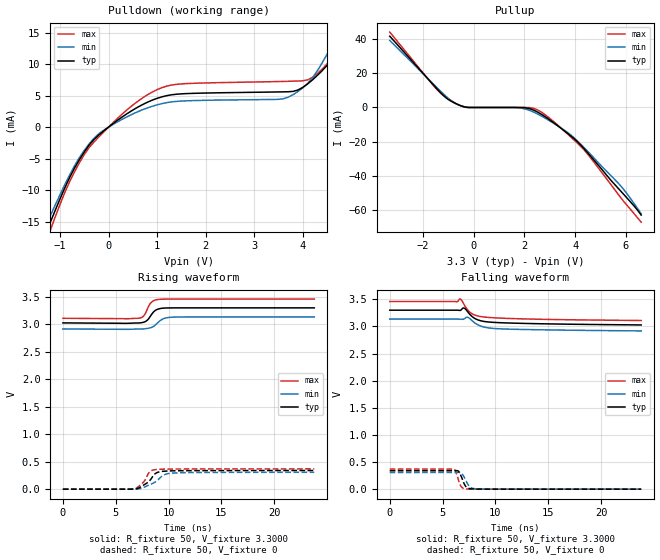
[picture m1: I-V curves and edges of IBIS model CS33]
|   IBIS Models For TG-5511CA (ClippedSine)
[IBIS Ver]   3.2
[File name]   tg5511ca_cs.ibs
[File Rev]   1.0
[Date]   Dec 3, 2020
[Source]   From silicon level SPICE model at Seiko Epson.
[Notes]
[Disclaimer]
This information is for modeling purposes only, and is not guaranteed.
Property of SEIKO EPSON Corp.,
unauthorized reproduction and/or distribution is strictly prohibited.
[Copyright]   Copyright 2020, SEIKO EPSON Corp. All rights reserved.
[Component]   TG-5511CA (ClippedSine)
[Manufacturer] SEIKO EPSON Corp.
[Package]
| variable   typ   min   max
R_pkg   99.0m   NA   NA
L_pkg   3.29n   NA   NA
C_pkg   0.40p   NA   NA
[Pin] signal_name   model_name   R_pin  L_pin  C_pin
  2   GND   GND   NA   NA   NA
  3   OUT   CS33   NA   NA   NA
  4   VCC   POWER   NA   NA   NA
| Models and submodels in the file (1): CS33 (Output)
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|   Model_type Output
[Model] CS33
Model_type  Output
Enable   Active-High
Polarity   Non-Inverting
Vmeas = 1.65
C_comp   2.5p   2.0p   3.0p
[Temperature Range]   25   85   -40
[Voltage Range]   3.3000   3.1350   3.4650
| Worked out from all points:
|   slope of the pulldown table from 0 to 0.495 V, typ, clamps not added: 184 ohm
|   falling waveform, R_fixture 50, V_fixture 3.3000: 20-80 % time 1.88ns typ, 2.1ns min, 1.61ns max; typ from 3.3 V to 3.03 V
|   falling waveform, R_fixture 50, V_fixture 0: 20-80 % time 453ps typ, 527ps min, 385ps max; typ from 0.34 V to 0 V
|   rising waveform, R_fixture 50, V_fixture 3.3000: 20-80 % time 675ps typ, 839ps min, 578ps max; typ from 3.03 V to 3.3 V
|   rising waveform, R_fixture 50, V_fixture 0: 20-80 % time 1.09ns typ, 1.46ns min, 815ps max; typ from 0 V to 0.34 V
[Pullup]
|   voltage I(typ)   I(min)   I(max)
-3.3V     41.62mA    39.12mA    44.01mA
-1.4V     10.28mA    11.01mA    9.827mA
-1.1V     5.864mA    6.748mA    6.095mA
-700mV    2.283mA    2.267mA    2.407mA
-300mV    152.5uA    251.6uA    75.7uA
1.8V      -4.05uA    -213.2uA   -94.5pA
2.3V      -1.159mA   -2.247mA   -272.4uA
2.8V      -5.195mA   -6.055mA   -4.027mA
3.7V      -15.1mA    -14.57mA   -15.44mA
4.2V      -21.6mA    -21.15mA   -22.42mA
5.8V      -48.88mA   -45.87mA   -52.72mA
6.6V      -62.82mA   -61.97mA   -66.95mA
[Pulldown]
|   voltage I(typ)   I(min)   I(max)
-3.3V     -61.57mA   -57.79mA   -65.45mA
-1.4V     -18.98mA   -17.58mA   -20.64mA
-1.2V     -15.12mA   -14.09mA   -16.38mA
-700mV    -6.498mA   -6.139mA   -7.097mA
-300mV    -1.962mA   -1.771mA   -2.366mA
1V        4.571mA    3.539mA    5.95mA
3.6V      5.603mA    4.498mA    7.258mA
4.2V      7.484mA    7.785mA    7.888mA
4.8V      13.35mA    15.8mA     12.77mA
5V        16.43mA    18.73mA    14.85mA
5.1V      18.03mA    20.21mA    16.09mA
6.6V      42.74mA    42.3mA     42.63mA
[Falling Waveform]
R_fixture = 50
V_fixture = 3.3000
V_fixture_min = 3.1350
V_fixture_max = 3.4650
0s        3.3V       3.135V     3.46V
6.4ns     3.3V       3.135V     3.455V
6.7ns     3.297V     3.134V     3.505V
6.9ns     3.336V     3.131V     3.454V
7.1ns     3.333V     3.146V     3.384V
7.4ns     3.265V     3.168V     3.299V
7.7ns     3.199V     3.124V     3.245V
8.4ns     3.117V     3.024V     3.19V
9.4ns     3.082V     2.972V     3.166V
23.8ns    3.028V     2.918V     3.11V
[Falling Waveform]
R_fixture = 50
V_fixture = 0
V_fixture_min = 0
V_fixture_max = 0
0s        340mV      307.6mV    370mV
6.1ns     340.9mV    308.7mV    369.9mV
6.2ns     341mV      308.7mV    347.7mV
6.5ns     333mV      308.7mV    173.9mV
6.7ns     264.1mV    304.2mV    66.64mV
6.9ns     171.9mV    269.7mV    22.06mV
7.2ns     49.75mV    165.3mV    5.263mV
7.6ns     8.533mV    41.6mV     1.957mV
8.3ns     1.868mV    5.22mV     789.2uV
23.8ns    0V         219.5uV    0V
[Rising Waveform]
R_fixture = 50
V_fixture = 3.3000
V_fixture_min = 3.1350
V_fixture_max = 3.4650
0s        3.026V     2.916V     3.11V
7.2ns     3.025V     2.915V     3.112V
7.7ns     3.042V     2.918V     3.165V
8ns       3.077V     2.926V     3.278V
8.4ns     3.18V      2.944V     3.405V
8.7ns     3.246V     2.979V     3.44V
9.1ns     3.282V     3.05V      3.454V
9.7ns     3.297V     3.114V     3.459V
10.6ns    3.299V     3.132V     3.46V
23.8ns    3.3V       3.135V     3.46V
[Rising Waveform]
R_fixture = 50
V_fixture = 0
V_fixture_min = 0
V_fixture_max = 0
0s        0V         209.3uV    0V
6.8ns     2.89mV     1.108mV    7.05mV
7.1ns     15.1mV     4.335mV    37.67mV
7.7ns     80.6mV     36.24mV    142.7mV
8.2ns     150.5mV    79.35mV    311.2mV
8.6ns     254.8mV    114.1mV    350.9mV
8.9ns     300.5mV    150.7mV    358.3mV
9.6ns     327mV      262.1mV    364.4mV
10.6ns    334.3mV    294.6mV    366.7mV
23.8ns    340mV      307.4mV    370mV
[Ramp]
| variable   typ   min   max
dV/dt_r   200.6m/1.094n   185.3m/1.468n   215.2m/0.819n
dV/dt_f   200.6m/0.455n   185.3m/0.53n   215.2m/0.387n
R_load = 50ohms
